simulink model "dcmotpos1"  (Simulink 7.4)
settings: Solver=ode15s  StartTime=0.0  StopTime=.1  MaxStep=1e-3  RelTol=1e-3

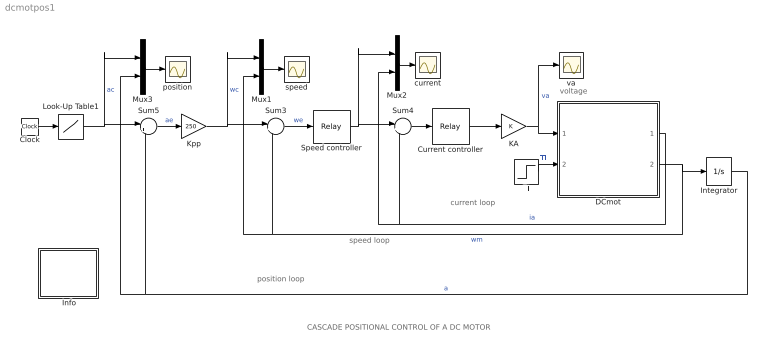
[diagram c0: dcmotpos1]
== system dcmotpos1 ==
  note: voltage
  note: speed loop
  note: current loop
  note: position loop
  note: CASCADE POSITIONAL CONTROL OF A DC MOTOR
  " Info" : Subsystem
  Clock : Clock
  Current controller : Relay  OnSwitchValue=0.5  OffSwitchValue=-0.5  OnOutputValue=60  OffOutputValue=-60  OutDataType=sfix(16)  OutScaling=2^0
  DCmot : Subsystem  mask{Ra=2.0, La=5.2e-3, J=1.5e-4, Bm=1e-3, K=0.1}
      mask prompts: Ra "Armature resistance [Ohm]"; La "Armature inductance [H]"; J "Moment of inertia [Kg.m^2]"; Bm "Frictional coefficient"; K "Electromechanical coupling coefficient"
      mask help: Block diagram representation of a dc motor
  Integrator : Integrator
  KA : Gain  ParameterDataType=sfix(16)  ParameterScaling=2^0  OutDataType=sfix(16)  OutScaling=2^0
  Kpp : Gain  Gain=250  ParameterDataType=sfix(16)  ParameterScaling=2^0  OutDataType=sfix(16)  OutScaling=2^0
  Look-Up Table1 : Lookup  InputValues="[0  .05  .05 1]"  Table="[1 1 .5  .5]"  OutDataType=sfix(16)  OutScaling=2^0
  Mux1 : Mux  Inputs=2
  Mux2 : Mux  Inputs=2
  Mux3 : Mux  Inputs=2
  Speed controller : Relay  OnSwitchValue=.025  OffSwitchValue=-.025  OnOutputValue=18  OffOutputValue=-18  OutDataType=sfix(16)  OutScaling=2^0
  Sum3 : Sum  Inputs=|+-  OutDataType=sfix(16)  OutScaling=2^0
  Sum4 : Sum  Inputs=|+-  OutDataType=sfix(16)  OutScaling=2^0
  Sum5 : Sum  Inputs=|+-  OutDataType=sfix(16)  OutScaling=2^0
  Tl : Step  Time=0.04  After=0.38  SampleTime=0
  current : Scope
  position : Scope
  speed : Scope
  va : Scope
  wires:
  Tl/1 -> DCmot/2(Tl)  "Tl"
  Mux1/1 -> speed/1
  Mux2/1 -> current/1
  Kpp/1 -> Sum3/1, Mux1/1  "wc"
  DCmot/1(ia) -> Sum4/2, Mux2/2  "ia"
  Sum5/1 -> Kpp/1  "ae"
  Clock/1 -> Look-Up Table1/1
  Mux3/1 -> position/1
  Look-Up Table1/1 -> Sum5/1, Mux3/1  "ac"
  Integrator/1 -> Sum5/2, Mux3/2  "a"
  Speed controller/1 -> Sum4/1, Mux2/1
  Sum3/1 -> Speed controller/1  "we"
  Sum4/1 -> Current controller/1
  KA/1 -> va/1, DCmot/1(va)  "va"
  DCmot/2(wm) -> Integrator/1, Sum3/2, Mux1/2  "wm"
  Current controller/1 -> KA/1

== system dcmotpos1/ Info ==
  note: This demo simulates the cascade control of a DC motor drive for position control

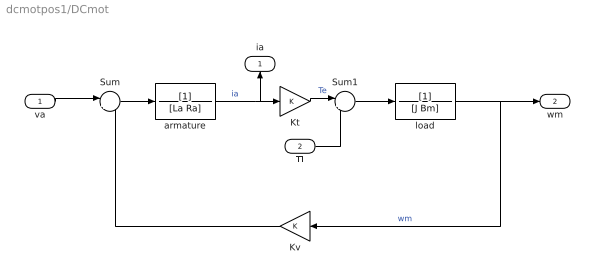
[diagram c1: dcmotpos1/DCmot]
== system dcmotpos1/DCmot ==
  va : Inport  OutDataType=sfix(16)  OutScaling=2^0
  Tl : Inport  Port=2  OutDataType=sfix(16)  OutScaling=2^0
  Kt : Gain  Gain=K  ParameterDataType=sfix(16)  ParameterScaling=2^0  OutDataType=sfix(16)  OutScaling=2^0
  Kv : Gain  Gain=K  ParameterDataType=sfix(16)  ParameterScaling=2^0  OutDataType=sfix(16)  OutScaling=2^0
  Sum : Sum  Inputs=|+-  OutDataType=sfix(16)  OutScaling=2^0
  Sum1 : Sum  Inputs=|+-  OutDataType=sfix(16)  OutScaling=2^0
  armature : TransferFcn  Denominator=[La Ra]
  load : TransferFcn  Denominator=[J Bm]
  ia : Outport
  wm : Outport  Port=2
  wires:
  Kt/1 -> Sum1/1  "Te"
  Tl/1 -> Sum1/2
  armature/1 -> Kt/1, ia/1  "ia"
  Sum1/1 -> load/1
  load/1 -> wm/1, Kv/1  "wm"
  Kv/1 -> Sum/2
  va/1 -> Sum/1
  Sum/1 -> armature/1
